ORGANIZATION_BLOCK MAIN:OB1
TITLE=Cancello elettrico automatico
//Simulatore: 09
//Versione: 1.0
//Data: 28/08/2002
//------------ Descrizione dell'impianto --------------------
//L'apertura e la chiusura di un cancello sono gestite dal
//motore M1 protetto dal relè termico FR.
//La posizione del cancello viene rilevata mediante due
//finecorsa SQ1 (cancello aperto) SQ2 (cancello chiuso).
//Per la sicurezza antiinfortunistica sono previste:
// - una fotocellula B che rileva l'interposizione fra
//   proiettore e ricevitore,
// - una costa pneumatica, posta nella parte fissa del
//   cancello che interviene nel caso di un'azione di
//   esterna di opposizione al movimento di chiusura
//   del cancello.
//
//L'apertura del cancello viene comandata dal pulsante SB1
//o dal pulsante SB2 del radiocomando, il pulsante SB3 può
//arrestare in qualsiasi momento l'apertura o la chiusura
//del cancello.
//Una volta avviata e completata l'apertura il cancello
//resterà nella posizione aperto per un certo tempo quindi
//verrà richiuso automaticamente.
//Durante la richiusura se interviene una delle due sicurezze
//il cancello verrà forzato in riapertura.
//Il comando del cancello può essere effetuata anche con il
//selettore a chiave SA che nella posizione 2 effetua
//l'apertura e nella posizione 1 la chiusura del cancello.
//
//La fase di movimentazione viene segnalata da un lampeggiatore
//HL4 (il lampeggio deve essere gestito dal PLC).
//Nel caso di intervento del termico FR il motore M1 verrà
//arrestato e la lampada HL2 segnalerà l'intervento della
//protezione.
//La lampada HL1 segnala invece lo stato ON-OFF del motore M1.
//

BEGIN
NETWORK 1 //Apertura cancello
//
LD I1.1 //P_SB1
O I1.2 //P_SB2
O I1.0 //S_SB4_2
ON I0.6 //SQ3
O I0.1 //B
O M1.0 //Marker Apertura
A I0.5 //FR
AN I0.7 //S_SB4_1
AN M1.1 //Marker Chiusura
A I0.0 //SQ1
A I1.3 //P_SB3
= M1.0 //Marker apertura

NETWORK 2 //Temporizzatore apertura
//
LDN I0.0 //SQ1
A I0.2 //SQ2
A I0.5 //FR
TON T37 +50
= M0.0 //Marker Aperto

NETWORK 3 //Chiusura cancello
//
LD T37
O M1.1 //Marker Chiusura
O I0.7 //S_SB4_1
AN M1.0 //Marker Apertura
AN I1.0 //S_SB4_2
A I0.6 //SQ3
A I0.2 //SQ2
A I0.5 //FR
AN I0.1 //B
A I1.3 //P_SB3
= M1.1 //Marker Chiusura

NETWORK 4 //Azionamento in apertura
//
LD M1.0 //Marker Apertura
AN I0.3 //KM2
= Q0.3

NETWORK 5 //Azionamento in chiusura
//
LD M1.1 //Marker Chiusura
AN I0.4 //KM1
= Q0.2 //VacB
= Q0.0

NETWORK 6 //Segnalazione Ciclo ON
//
LD M1.0 //Marker Apertura
O M1.1 //Marker Chiusura
O M0.0 //Marker Aperto
= Q0.6 //HL3

NETWORK 7 //Lampeggio Lampada Movimento
//
LD SM0.5 //
A Q0.6 //HL3
= Q0.1 //HL4

NETWORK 8 //Segnalazione relè termico scattato
//
LDN I0.5 //FR
= Q0.5 //HL2

NETWORK 9 //Segnalazione Motore ON
//
LD Q0.2 //KM1
O Q0.3 //KM2
= Q0.4 //HL1

END_ORGANIZATION_BLOCK

